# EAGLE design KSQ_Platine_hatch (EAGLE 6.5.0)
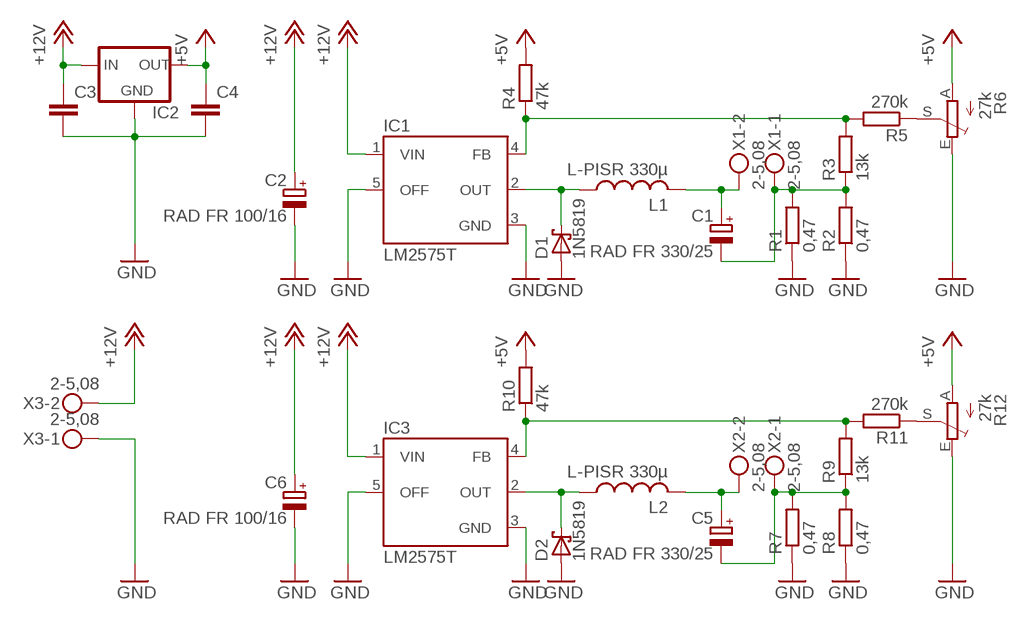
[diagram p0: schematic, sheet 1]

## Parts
C1  RAD FR 330/25  CPOL-EUE3.5-8  [E3,5-8]
C2  RAD FR 100/16  CPOL-EUE2-5  [E2-5]
C3  C-EUC0805  [C0805]
C4  C-EUC0805  [C0805]
C5  RAD FR 330/25  CPOL-EUE3.5-8  [E3,5-8]
C6  RAD FR 100/16  CPOL-EUE2-5  [E2-5]
D1  1N5819  1N5819-T  [DO41-7.6]
D2  1N5819  1N5819-T  [DO41-7.6]
IC1  LM2575T  [TO220-5]
IC2  78LXX  [78LXX]
IC3  LM2575T  [TO220-5]
L1  L-PISR 330µ  L-USPISR  [PISR]
L2  L-PISR 330µ  L-USPISR  [PISR]
R1  0,47  R-EU_0207/10  [0207/10]
R2  0,47  R-EU_0207/10  [0207/10]
R3  13k  R-EU_0207/10  [0207/10]
R4  47k  R-EU_0207/10  [0207/10]
R5  270k  R-EU_0207/10  [0207/10]
R6  27k  TRIM_EU-CA6V  [CA6V]
R7  0,47  R-EU_0207/10  [0207/10]
R8  0,47  R-EU_0207/10  [0207/10]
R9  13k  R-EU_0207/10  [0207/10]
R10  47k  R-EU_0207/10  [0207/10]
R11  270k  R-EU_0207/10  [0207/10]
R12  27k  TRIM_EU-CA6V  [CA6V]
X1  2-5,08  MKDSN1,5/2-5,08  [MKDSN1,5/2-5,08]
X2  2-5,08  MKDSN1,5/2-5,08  [MKDSN1,5/2-5,08]
X3  2-5,08  MKDSN1,5/2-5,08  [MKDSN1,5/2-5,08]

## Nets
+5V: C4.1 IC2.OUT R4.2 R6.A R10.2 R12.A
+12V: C2.+ C3.1 C6.+ IC1.1(VIN) IC2.IN IC3.1(VIN) X3.2
GND: C2.- C3.2 C4.2 C6.- D1.A D2.A IC1.3(GND) IC1.5(OFF) IC2.GND IC3.3(GND) IC3.5(OFF) R1.1 R2.1 R6.E R7.1 R8.1 R12.E X3.1
N$1: D1.C IC1.2(OUT) L1.1
N$2: C1.+ L1.2 X1.2
N$3: C1.- R1.2 R2.2 R3.1 X1.1
N$4: IC1.4(FB) R3.2 R4.1 R5.2
N$5: R5.1 R6.S
N$6: D2.C IC3.2(OUT) L2.1
N$7: C5.+ L2.2 X2.2
N$8: C5.- R7.2 R8.2 R9.1 X2.1
N$9: IC3.4(FB) R9.2 R10.1 R11.2
N$10: R11.1 R12.S

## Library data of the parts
C1 C2 C5 C6 = rcl:CPOL-EU: POLARIZED CAPACITOR, European symbol
C3 C4 = rcl:C-EU: CAPACITOR, European symbol
D1 D2 = diode:1N581*: 1.0A SCHOTTKY BARRIER RECTIFIER
IC1 IC3 = v-reg-3:LM2575: National Semiconductor 1.0A "Simple Switcher"(c) 52kHz, Vout 1.23-37V (HV: 57V), Vin 40V (HV: 60V), 50µA standby current
IC2 = v-reg:78LXX: VOLTAGE REGULATOR
L1 L2 = Inductor-Fastron:L-US
R1-R5 R7-R11 = rcl:R-EU_: RESISTOR, European symbol
R6 R12 = pot:TRIM_EU-: POTENTIOMETER
X1-X3 = con-phoenix-508:MKDSN1,5/2-5,08: MKDSN 1,5/ 2-5,08 Printklemme; MPN: MKDSN 1,5/2-5.08; OC_FARNELL: 1792903; OC_NEWARK: 30M2397

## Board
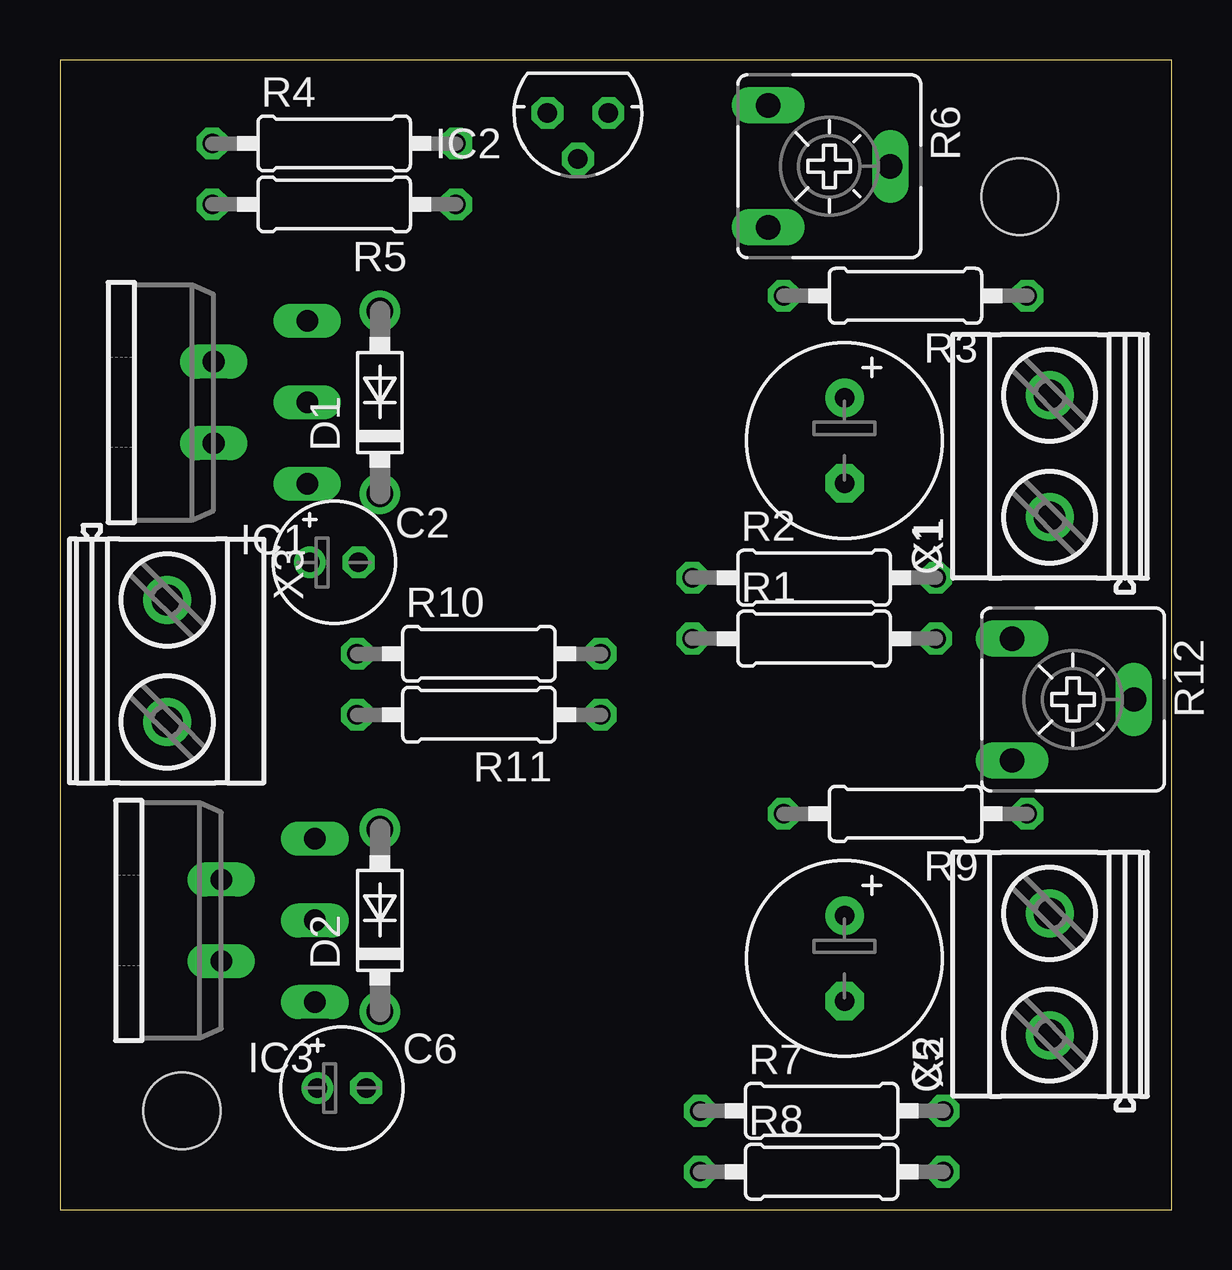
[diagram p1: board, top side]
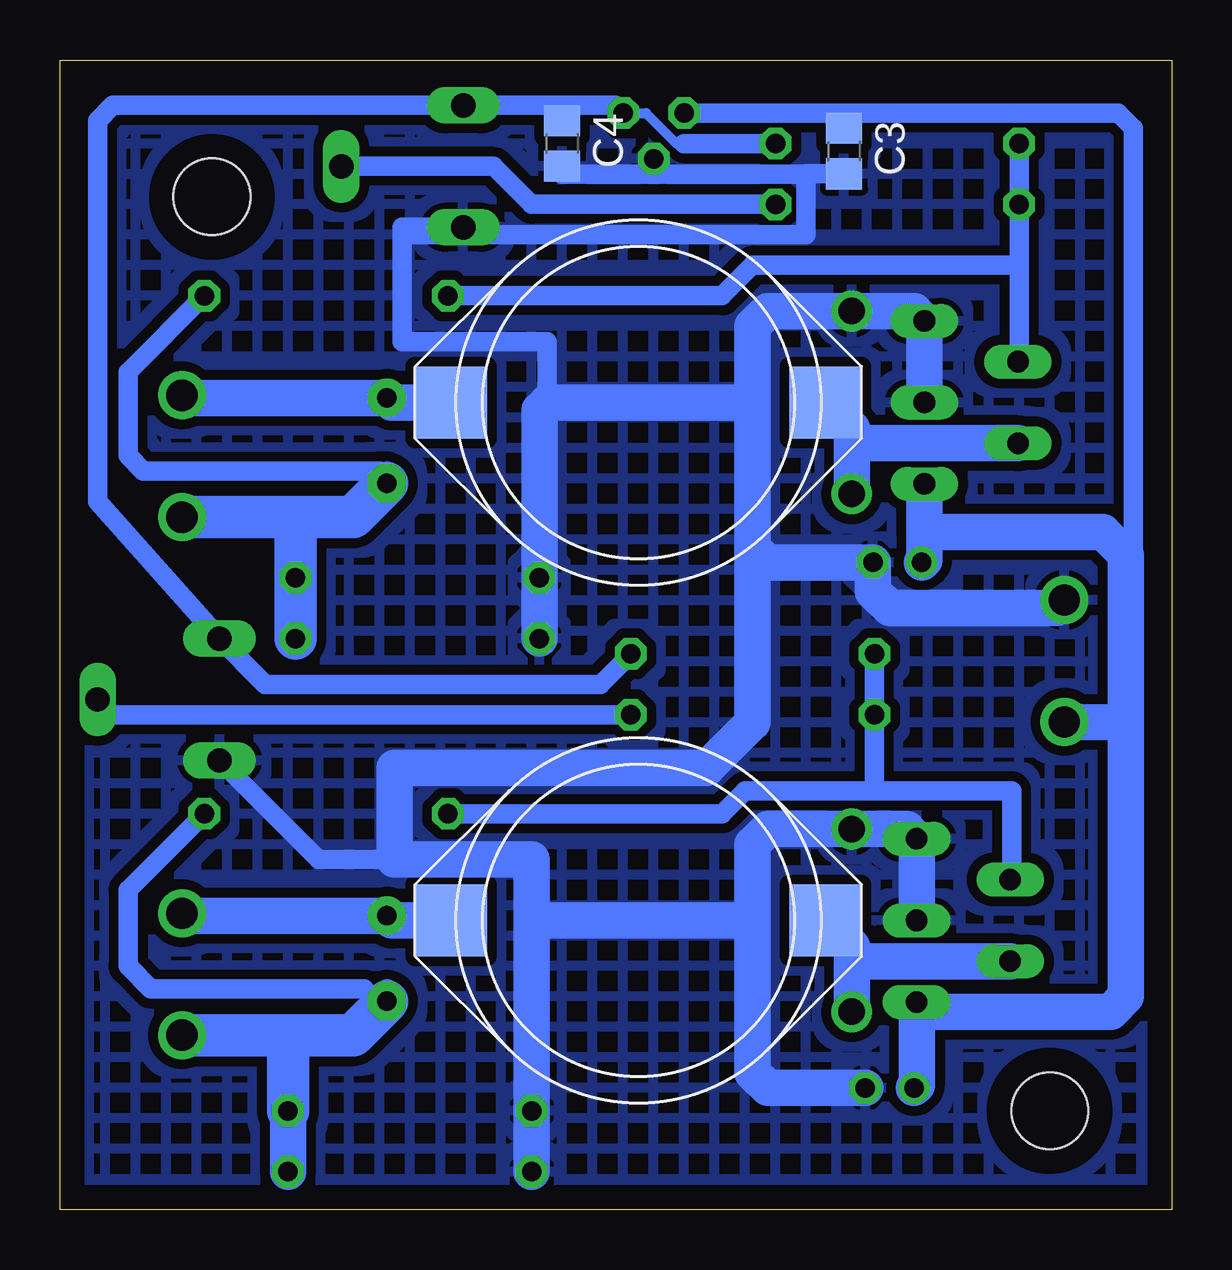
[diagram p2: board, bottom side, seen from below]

Size 46.34 x 47.93 mm. Coordinates in mm from the lower left corner, seen from the top.
Outline: 0,0 46.34,0 46.34,47.93 0,47.93 0,0
Copper layers (1*16): Top 0.035mm / dielectric 1.5mm / Bottom 0.035mm
Design rules "default": minimum track width 10mil, minimum drill 24mil, track to track 8mil, track to pad 8mil, pad to pad 8mil, via to via 8mil, smd to smd 8mil, copper to edge 40mil, drill to drill 8mil, minimum pad ring 10mil, minimum via ring 8mil, stop-mask expansion 4mil, vias tented up to drill 0mil, thermal gap 10mil
Holes 3.2 mm at 40.01,42.23 5.08,4.13

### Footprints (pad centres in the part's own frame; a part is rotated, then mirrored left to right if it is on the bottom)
E3,5-8 = drill 0.813 pad 1.6: + -1.778,0 | drill 0.813 pad 1.6 octagon: - 1.778,0
E2-5 = drill 0.813 pad 1.27: + -1.016,0 | drill 0.813 pad 1.27 octagon: - 1.016,0
C0805 = smd 1.3 x 1.5: 1 -0.95,0; 2 0.95,0
DO41-7.6 = drill 1.1 pad 1.7: A 3.81,0; C -3.81,0
TO220-5 = drill 0.9 long: 1 -3.4,-8.4; 2 -1.7,-4.5; 3 0,-8.4; 4 1.7,-4.5; 5 3.4,-8.4
78LXX = drill 0.813 octagon: GND 0,1.905; IN 1.27,0; OUT -1.27,0
PISR = smd 3 x 3: 1 -7.8,0; 2 7.8,0
0207/10 = drill 0.813 octagon: 1 -5.08,0; 2 5.08,0
CA6V = drill 1.016 long: A -2.54,-2.54; E 2.54,-2.54; S 0,2.54
MKDSN1,5/2-5,08 = drill 1.3 pad 2: 1 -2.561,0.025; 2 2.519,0.025

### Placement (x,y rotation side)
C1  32.7,32.07 270 top
C2  11.43,26.99 0 top
C3  13.65,44.13 270 bottom
C4  25.4,44.45 270 bottom
C5  32.7,10.48 270 top
C6  11.75,5.08 0 top
D1  13.34,33.66 90 top
D2  13.34,12.06 90 top
IC1  1.91,33.66 90 top
IC2  21.59,45.72 180 top
IC3  2.22,12.06 90 top
L1  22.23,33.66 180 bottom
L2  22.23,12.06 180 bottom
R1  31.43,23.81 0 top
R2  31.43,26.35 0 top
R3  35.24,38.1 180 top
R4  11.43,44.45 0 top
R5  11.43,41.91 180 top
R6  32.07,43.5 270 top
R7  31.75,4.13 0 top
R8  31.75,1.59 0 top
R9  35.24,16.51 180 top
R10  17.46,23.18 0 top
R11  17.46,20.64 180 top
R12  42.23,21.27 270 top
X1  41.27,31.43 90 top
X2  41.27,9.84 90 top
X3  4.45,22.86 270 top

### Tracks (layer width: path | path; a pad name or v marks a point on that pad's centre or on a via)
+5V
  Bottom 0.406: 20.32,44.45 20.64,44.45 21.91,45.72 IC2.OUT
  Bottom 0.813: 20.32,44.45 R4.2 | IC2.OUT 23.18,46.04 25.4,46.04 | 25.4,46.04 R6.A 44.13,46.04 44.77,45.4 44.77,29.53 R12.A 37.78,21.91 23.81,21.91 R10.2 | 25.4,46.04 C4.1
+12V
  Bottom 0.813: 10.3,30.02 IC1.1 | 10.62,8.08 IC3.1 | 13.65,45.72 2.22,45.72 1.59,45.09 1.59,27.3 1.91,26.99 | 13.65,45.72 IC2.IN | 13.65,45.72 C3.1
  Bottom 1.524: 10.3,28.26 10.3,30.02 | 10.3,28.26 10.3,27.1 C2.+ | 10.62,7.94 10.62,5.19 C6.+ | 10.62,7.94 10.62,8.08 | 1.91,20.32 1.91,26.99 1.91,27.3 2.86,28.26 10.3,28.26 | X3.2 3.83,20.34 1.91,20.32 | 1.91,20.32 1.91,8.89 2.54,8.26 10.3,8.26 10.62,7.94
GND
  Bottom 0.813: 10.3,34.12 IC1.3 | 26.04,33.66 26.04,36.2 32.07,36.2 32.07,40.64 | R6.E 32.07,40.96 32.07,40.64 | IC2.GND 21.59,43.5 21.27,43.18 | 15.24,43.18 21.27,43.18 | 15.24,43.18 15.24,40.64 32.07,40.64 | C3.2 15.24,43.18 | C4.2 25.4,43.18 21.27,43.18 | 10.62,12.53 IC3.3 | R12.E 35.56,14.61 32.38,14.61
  Bottom 1.524: 10.3,34.12 IC1.5 10.71,37.47 D1.A 16.83,37.47 17.46,36.83 17.46,33.97 | 17.46,33.97 17.78,33.66 26.04,33.66 26.35,33.34 R2.1 R1.1 | 17.46,27.62 16.83,26.99 C2.- 12.45,25.78 11.75,25.08 4.81,25.08 X3.1 | 17.46,27.62 17.46,33.97 | 10.62,12.53 IC3.5 11.03,15.88 D2.A 16.83,15.88 17.46,15.24 17.46,12.06 | 17.46,12.06 26.67,12.06 | C6.- 16.83,5.08 17.46,5.71 17.46,12.06 | R8.1 R7.1 26.67,12.06 | 26.67,12.06 26.67,14.61 32.38,14.61 32.38,18.41 19.37,18.41 17.46,20.32 17.46,27.62
  pour Bottom (isolate 0.406, hatched): 0,47.94 46.35,47.94 46.35,0 0,0
N$1
  Bottom 1.524: 13.34,32.07 D1.C | 13.34,32.07 13.34,32.56 L1.1 | IC1.2 13.22,31.95 13.34,32.07
N$2
  Bottom 1.524: L1.2 32.51,33.66 C1.+ 41.14,33.85 X1.2
N$3
  Bottom 0.813: R3.1 43.5,34.92 43.5,31.43 42.86,30.8 33.02,30.8 32.7,30.48 | C1.- 32.7,30.48 | 32.7,30.48 32.7,30.8
  Bottom 1.778: X1.1 36.51,28.87 | 36.51,28.87 34.12,28.87 C1.- | R1.2 R2.2 36.51,28.87
N$4
  Bottom 0.813: R3.2 18.73,38.1 17.46,39.37 6.35,39.37 | 6.35,39.37 6.35,35.41 IC1.4 | R4.1 R5.2 6.35,39.37
N$5
  Bottom 0.813: R5.1 26.67,41.91 28.26,43.5 R6.S
N$6
  Bottom 1.524: 13.34,10.48 D2.C | 13.34,10.48 13.34,10.97 L2.1 | IC3.2 13.22,10.37 13.34,10.48
N$7
  Bottom 1.524: L2.2 32.51,12.06 C5.+ 41.14,12.26 X2.2
N$8
  Bottom 0.813: R9.1 43.5,13.34 43.5,10.16 42.55,9.21 33.66,9.21 33.34,8.89 32.7,8.89 | C5.- 32.7,8.89 | 32.7,9.21 32.7,8.89
  Bottom 1.524: R8.2 R7.2
  Bottom 1.778: X2.1 36.83,7.28 | 36.83,7.28 34.12,7.28 C5.- | R7.2 36.83,7.28
N$9
  Bottom 0.813: R9.2 18.73,16.51 17.78,17.46 12.38,17.46 | 12.38,17.46 6.67,17.46 6.67,13.82 IC3.4 | R10.1 R11.2 12.38,17.46
N$10
  Bottom 0.813: R11.1 44.13,20.64 R12.S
